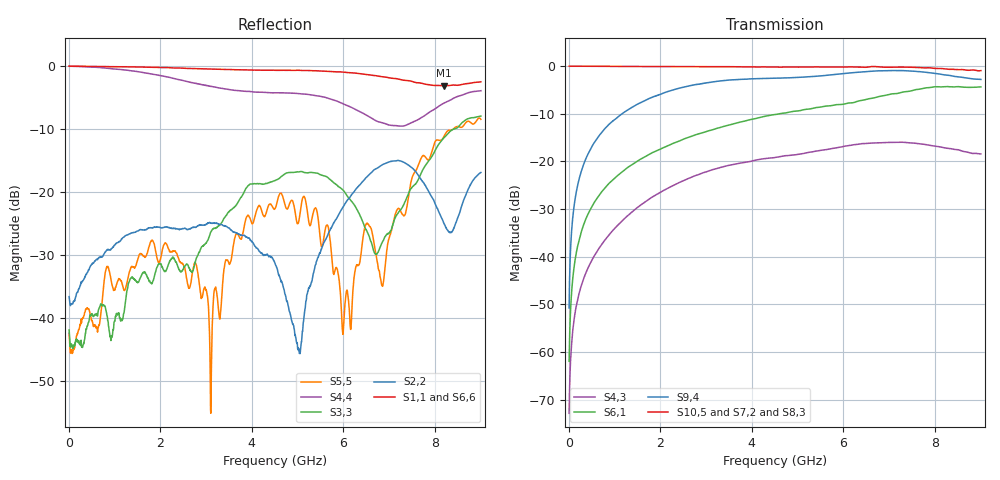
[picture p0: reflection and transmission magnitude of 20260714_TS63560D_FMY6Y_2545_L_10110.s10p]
# GHz S DB R 50
! CMT, SN0916, 25263762, 26.7.0
! Date: 15.07.2026 13:45:37
! Data: Format
! Freq S1.1:dB/Ang S1.2:dB/Ang S1.3:dB/Ang S1.4:dB/Ang S1.5:dB/Ang S1.6:dB/Ang S1.7:dB/Ang S1.8:dB/Ang S1.9:dB/Ang S1.10:dB/Ang
!  S2.1:dB/Ang S2.2:dB/Ang S2.3:dB/Ang S2.4:dB/Ang S2.5:dB/Ang S2.6:dB/Ang S2.7:dB/Ang S2.8:dB/Ang S2.9:dB/Ang S2.10:dB/Ang
!  S3.1:dB/Ang S3.2:dB/Ang S3.3:dB/Ang S3.4:dB/Ang S3.5:dB/Ang S3.6:dB/Ang S3.7:dB/Ang S3.8:dB/Ang S3.9:dB/Ang S3.10:dB/Ang
!  S4.1:dB/Ang S4.2:dB/Ang S4.3:dB/Ang S4.4:dB/Ang S4.5:dB/Ang S4.6:dB/Ang S4.7:dB/Ang S4.8:dB/Ang S4.9:dB/Ang S4.10:dB/Ang
!  S5.1:dB/Ang S5.2:dB/Ang S5.3:dB/Ang S5.4:dB/Ang S5.5:dB/Ang S5.6:dB/Ang S5.7:dB/Ang S5.8:dB/Ang S5.9:dB/Ang S5.10:dB/Ang
!  S6.1:dB/Ang S6.2:dB/Ang S6.3:dB/Ang S6.4:dB/Ang S6.5:dB/Ang S6.6:dB/Ang S6.7:dB/Ang S6.8:dB/Ang S6.9:dB/Ang S6.10:dB/Ang
!  S7.1:dB/Ang S7.2:dB/Ang S7.3:dB/Ang S7.4:dB/Ang S7.5:dB/Ang S7.6:dB/Ang S7.7:dB/Ang S7.8:dB/Ang S7.9:dB/Ang S7.10:dB/Ang
!  S8.1:dB/Ang S8.2:dB/Ang S8.3:dB/Ang S8.4:dB/Ang S8.5:dB/Ang S8.6:dB/Ang S8.7:dB/Ang S8.8:dB/Ang S8.9:dB/Ang S8.10:dB/Ang
!  S9.1:dB/Ang S9.2:dB/Ang S9.3:dB/Ang S9.4:dB/Ang S9.5:dB/Ang S9.6:dB/Ang S9.7:dB/Ang S9.8:dB/Ang S9.9:dB/Ang S9.10:dB/Ang
!  S10.1:dB/Ang S10.2:dB/Ang S10.3:dB/Ang S10.4:dB/Ang S10.5:dB/Ang S10.6:dB/Ang S10.7:dB/Ang S10.8:dB/Ang S10.9:dB/Ang S10.10:dB/Ang
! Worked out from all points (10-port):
!   2001 points, 10 MHz to 9 GHz, reference 50 ohm
!   strongest paths, dB at 10 MHz, 2.257 GHz, 4.505 GHz, 6.753 GHz, 9 GHz:
!     S10,5: -0.1, -0.2, -0.2, -0.2, -1.0
!     S7,2: -0.1, -0.2, -0.3, -0.6, -0.6
!     S8,3: -0.1, -0.2, -0.4, -0.4, -1.2
!     S9,4: -50.8, -5.1, -2.6, -1.1, -2.8
!     S6,1: -62.0, -16.4, -10.2, -6.5, -4.4
!     S4,3: -72.9, -25.2, -19.2, -16.2, -18.5
!   lowest |S11| = -3.1 dB at 8.2 GHz (marker M1), VSWR 5.61, Z = 11.1 - j24.1 ohm
!   |S11| at or under -10 dB: nowhere
